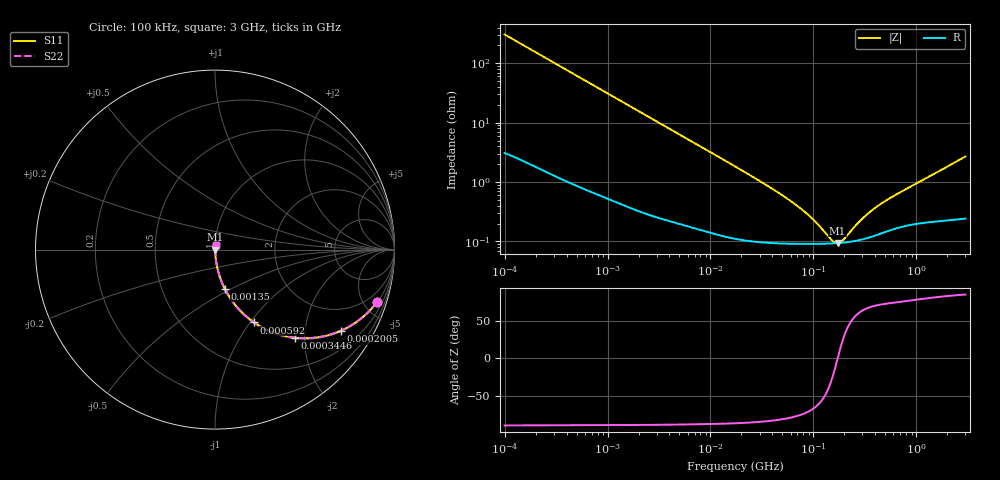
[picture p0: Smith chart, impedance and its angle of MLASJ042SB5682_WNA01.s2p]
! MLASJ042SB5682_WNA01  S-PARAMETER MODEL  ( Standard Model )
! Model Generated by TAIYO YUDEN Corporation (http://www.ty-top.com)
! Version 1.0
! TAIYO YUDEN Control No. 220601
! Copyright(c) 2007 TAIYO YUDEN CO.,LTD. All Rights Reserved.
! Product Description (link to TY-COMPAS)
! https://ds.yuden.co.jp/TYCOMPAS/or/detail?pn=MLASJ042SB5682KWNA01&u=M
! Products Name : Multilayer Ceramic Capacitors
! Characteristics :
!  Capacitance : 6800 [pF] , Rated Voltage : 6.3 [V] , TCC : X5R
!  Case Size : 0.4 x 0.2 / 0.016 x 0.008 [mm/inch] , Thickness : 0.2 / 0.008 [mm/inch]
!  (Conditions: Temperature = 25 [degC] , DC Bias Voltage = 0 [V])
! External Node Assignments :
!  1  o---| |---o  2
! GND o---------o GND
! Frequency Range : 100kHz  -  3GHz  [ 401 STEP ]
# MHZ S RI R 50
! Freq[MHz].  S11 Real  S11 Imag  S21 Real  S21 Imag  S12 Real  S12 Imag  S22 Real  S22 Imag
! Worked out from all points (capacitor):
!   401 points, 100 kHz to 3 GHz, reference 50 ohm
!   read as one part in series: C = 5.2 nF near 105.3 kHz
!   lowest |Z| = 94 mohm at 171.7 MHz (marker M1)
!   series resonance near 172.2 MHz, so ESL is about 160 pH
!   S11 on the Smith chart (normalised r, x): 100 kHz: 1.06, -6.11; 200.5 kHz: 1.04, -3.07; 344.6 kHz: 1.02, -1.79; 592 kHz: 1.02, -1.05; 1.35 MHz: 1.01, -0.46; 3 GHz: 1.00, +0.05
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0.1  0.901 -0.2937  0.099 0.2937  0.099 0.2937  0.901 -0.2937
0.1398  0.8251 -0.3744  0.1749 0.3744  0.1749 0.3744  0.8251 -0.3744
0.200542  0.6993 -0.4528  0.3007 0.4528  0.3007 0.4528  0.6993 -0.4528
0.266273  0.5714 -0.4888  0.4286 0.4888  0.4286 0.4888  0.5714 -0.4888
0.344552  0.4458 -0.4907  0.5542 0.4907  0.5542 0.4907  0.4458 -0.4907
0.562235  0.236 -0.4175  0.764 0.4175  0.764 0.4175  0.236 -0.4175
0.591975  0.2184 -0.406  0.7816 0.406  0.7816 0.406  0.2184 -0.406
0.871356  0.1169 -0.3132  0.8831 0.3132  0.8831 0.3132  0.1169 -0.3132
1.350433  0.0543 -0.2176  0.9457 0.2176  0.9457 0.2176  0.0543 -0.2176
3.161081  0.0122 -0.0981  0.9878 0.0981  0.9878 0.0981  0.0122 -0.0981
6.674626  0.00395 -0.0473  0.996 0.0473  0.996 0.0473  0.00395 -0.0473
17.7727  0.00142 -0.0179  0.9986 0.0179  0.9986 0.0179  0.00142 -0.0179
52.46276  0.000952 -0.00558  0.999 0.00558  0.999 0.00558  0.000952 -0.00558
73.34282  0.000923 -0.0036  0.9991 0.0036  0.9991 0.0036  0.000923 -0.0036
97.38194  0.000915 -0.00226  0.9991 0.00226  0.9991 0.00226  0.000915 -0.00226
150.9232  0.000927 -0.000497  0.9991 0.000497  0.9991 0.000497  0.000927 -0.000497
171.6802  0.000939 -1.09e-05  0.9991 1.09e-05  0.9991 1.09e-05  0.000939 -1.09e-05
195.2919  0.000957 0.000475  0.999 -0.000475  0.999 -0.000475  0.000957 0.000475
266.0711  0.00104 0.00168  0.999 -0.00168  0.999 -0.00168  0.00104 0.00168
335.5313  0.00115 0.00267  0.9989 -0.00267  0.9989 -0.00267  0.00115 0.00267
547.5153  0.00155 0.00506  0.9984 -0.00506  0.9984 -0.00506  0.00155 0.00506
3000  0.00314 0.0267  0.9969 -0.0267  0.9969 -0.0267  0.00314 0.0267
